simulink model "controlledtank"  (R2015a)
settings: Solver=ode45  StartTime=0.0  StopTime=50.0  RelTol=1e-3

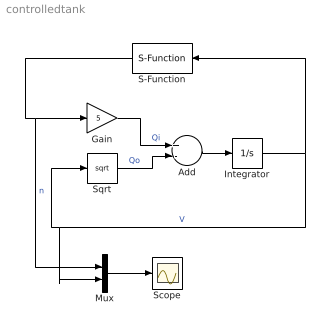
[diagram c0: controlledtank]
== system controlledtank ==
  Add : Sum  Inputs=+-
  Gain : Gain  Gain=5
  Integrator : Integrator
  Mux : Mux  Inputs=2
  S-Function : S-Function  FunctionName=tank_ctrl
  Scope : Scope
  Sqrt : Sqrt
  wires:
  Add/1 -> Integrator/1
  Sqrt/1 -> Add/2  "Qo"
  S-Function/1 -> Gain/1, Mux/1  "n"
  Gain/1 -> Add/1  "Qi"
  Mux/1 -> Scope/1
  Integrator/1 -> Sqrt/1, Mux/2, S-Function/1  "V"
